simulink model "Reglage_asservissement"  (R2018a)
settings: Solver=FixedStepAuto  StartTime=0.0  StopTime=inf  RelTol=1e-3  EnableMultiTasking=on
libraries: arduinolib x3, simulink x2

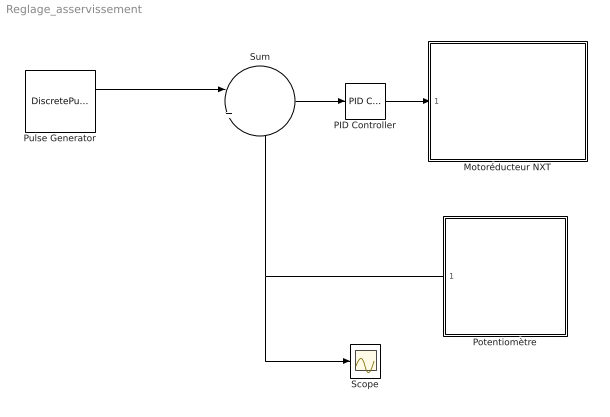
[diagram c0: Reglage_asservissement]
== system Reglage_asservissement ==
  Motoréducteur NXT : Subsystem
  PID Controller : simulink/Continuous/PID Controller  Controller=PID  TimeDomain=Discrete-time  SampleTime=-1  IntegratorMethod=Forward Euler  FilterMethod=Forward Euler  Form=Parallel  UseFilter=on  ControllerParametersSource=internal  P=0.3  I=0  D=0.025  N=100  InitialConditionSource=internal  InitialConditionForIntegrator=0  InitialConditionForFilter=0  ExternalReset=none  LimitOutput=off  UpperSaturationLimit=inf  LowerSaturationLimit=-inf  LinearizeAsGain=on  AntiWindupMode=none  Kb=1  TrackingMode=off  Kt=1  PParamMin=[]  PParamMax=[]  IParamMin=[]  IParamMax=[]  DParamMin=[]  DParamMax=[]  NParamMin=[]  NParamMax=[]  KbParamMin=[]  KbParamMax=[]  KtParamMin=[]  KtParamMax=[]  POutMin=[]  POutMax=[]  IOutMin=[]  IOutMax=[]  DOutMin=[]  DOutMax=[]  NOutMin=[]  NOutMax=[]  KbOutMin=[]  KbOutMax=[]  KtOutMin=[]  KtOutMax=[]  IntegratorOutMin=[]  IntegratorOutMax=[]  FilterOutMin=[]  FilterOutMax=[]  SumOutMin=[]  SumOutMax=[]  SumI1OutMin=[]  SumI1OutMax=[]  SumI2OutMin=[]  SumI2OutMax=[]  SumI3OutMin=[]  SumI3OutMax=[]  SumDOutMin=[]  SumDOutMax=[]  SaturationOutMin=[]  SaturationOutMax=[]  IntegratorContinuousStateAttributes=''  IntegratorStateMustResolveToSignalObject=off  IntegratorRTWStateStorageClass=Auto  FilterContinuousStateAttributes=''  FilterStateMustResolveToSignalObject=off  FilterRTWStateStorageClass=Auto  DifferentiatorICPrevScaledInput=0  DifferentiatorOutMin=[]  DifferentiatorOutMax=[]  FilterDiffOutCoefMin=[]  FilterDiffOutCoefMax=[]  SumDenOutMin=[]  SumDenOutMax=[]  SumNumOutMin=[]  SumNumOutMax=[]  ReciprocalOutMin=[]  ReciprocalOutMax=[]  DivideOutMin=[]  DivideOutMax=[]  TunerSelectOption=Transfer Function Based (PID Tuner App)
  Potentiomètre : Subsystem
  Pulse Generator : DiscretePulseGenerator  PulseType=Time based  Amplitude=90  PulseWidth=50
  Scope : Scope
  Sum : Sum  Inputs=|+-
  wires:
  Potentiomètre/1(Out1) -> Scope/1, Sum/2
  Sum/1 -> PID Controller/1
  PID Controller/1 -> Motoréducteur NXT/1(U)
  Pulse Generator/1 -> Sum/1

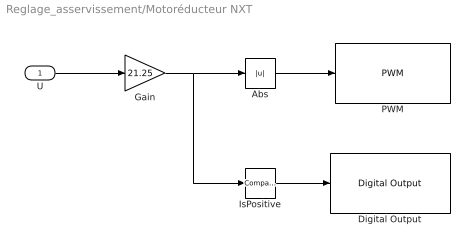
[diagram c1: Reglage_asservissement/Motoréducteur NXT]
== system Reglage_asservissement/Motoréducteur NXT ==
  U : Inport
  Abs : Abs
  Digital Output : arduinolib/Digital Output  pinNumber=12  blockPlatform=arduino
  Gain : Gain  Gain=21.25
  IsPositive : simulink/Logic and Bit Operations/Compare To Zero  relop=>  OutDataTypeStr=boolean
  PWM : arduinolib/PWM  pinNumber=3  EnableInputFrequency=off  InitialFrequency=2000  InitialDutyCycle=0  NotificationType=None  blockPlatform=arduino
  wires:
  IsPositive/1 -> Digital Output/1
  U/1 -> Gain/1
  Gain/1 -> IsPositive/1, Abs/1
  Abs/1 -> PWM/1

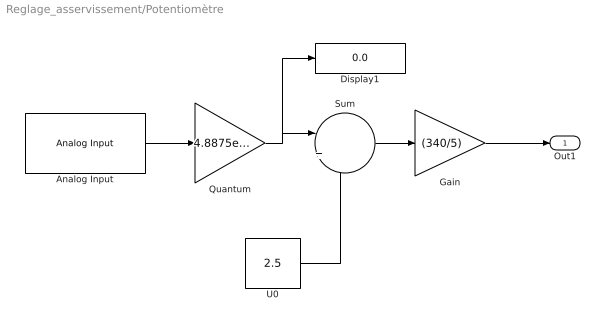
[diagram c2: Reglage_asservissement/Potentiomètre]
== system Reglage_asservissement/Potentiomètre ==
  Analog Input : arduinolib/Analog Input  pinNumber=5  ReadResultsOnly=off  ConversionTriggerSource=Software  ExternalTriggerType=uint32(0)  OutputDataType=uint16  EnableConversionCompleteNotify=off  EnableOuputStatus=off  SampleTime=0.01  blockPlatform=arduino
  Display1 : Display
  Gain : Gain  Gain=(340/5)
  Quantum : Gain  Gain=4.8875e-3
  Sum : Sum  Inputs=|+-
  U0 : Constant  Value=2.5
  Out1 : Outport
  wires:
  Gain/1 -> Out1/1
  Analog Input/1 -> Quantum/1
  Quantum/1 -> Display1/1, Sum/1
  U0/1 -> Sum/2
  Sum/1 -> Gain/1
